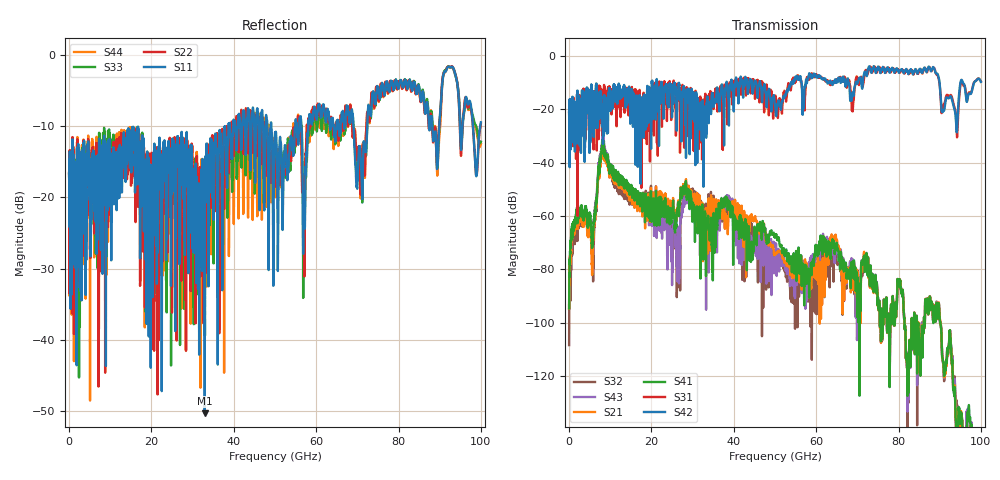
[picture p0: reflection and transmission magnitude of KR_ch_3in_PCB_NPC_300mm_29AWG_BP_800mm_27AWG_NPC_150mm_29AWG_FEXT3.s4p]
# GHz S RI R 45
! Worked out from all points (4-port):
!   4000 points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, 25 MHz to 100 GHz, reference 45 ohm
!   strongest paths, dB at 25 MHz, 25.02 GHz, 50.02 GHz, 75.03 GHz, 100 GHz:
!     S42: -21.2, -20.7, -18.6, -4.1, -9.8
!     S31: -21.3, -14.8, -15.7, -5.1, -9.6
!     S41: -94.6, -59.7, -67.7, -91.8, -144.8
!     S21: -94.8, -56.5, -74.3, -92.0, -149.7
!     S43: -94.5, -85.9, -72.0, -91.6, -151.6
!     S32: -108.3, -69.0, -77.0, -91.8, -151.4
!   lowest |S11| = -50.3 dB at 32.95 GHz (marker M1), VSWR 1.01, Z = 45 - j0.272 ohm
!   |S11| at or under -10 dB: start of sweep to 38.73 GHz; 49.11 GHz to 54.96 GHz (5.852 GHz wide, 11.2 % of centre); 69.03 GHz to 72.39 GHz (3.361 GHz wide, 4.75 % of centre)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
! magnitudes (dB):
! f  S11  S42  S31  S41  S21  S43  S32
! 25 MHz  -16.7  -21.2  -21.3  -94.6  -94.8  -94.5  -108.3
! 5.825 GHz  -14.5  -15.4  -17.4  -67.6  -70.3  -66.5  -81.0
! 8.25 GHz  -12.8  -33.0  -14.6  -31.9  -33.6  -30.6  -32.1
! 26.48 GHz  -15.0  -14.9  -12.1  -55.2  -54.9  -64.4  -66.4
! 28.6 GHz  -12.2  -13.1  -12.7  -54.0  -52.6  -55.2  -52.3
! 32.95 GHz  -50.3  -21.3  -24.4  -58.7  -60.8  -63.9  -66.6
! 100 GHz  -9.5  -9.8  -9.6  -144.8  -149.7  -151.6  -151.4
